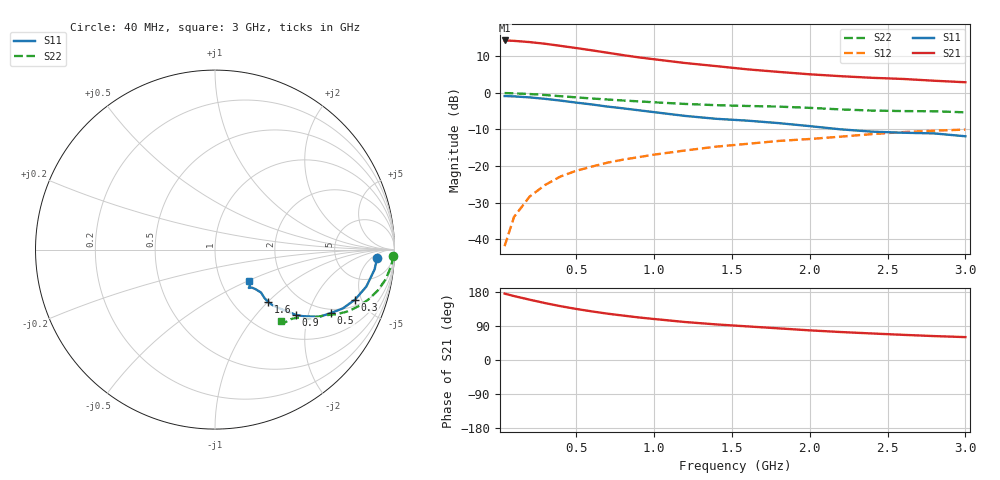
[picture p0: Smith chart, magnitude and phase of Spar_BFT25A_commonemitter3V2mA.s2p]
! Filename:  BFT25AJ.S2P  Version:  2.0
! NXP part #: BFT25A  Date: Aug 1990
! Bias condition: Vce=3V, Ic=2mA
#  MHz  S  MA  R  50
! Freq  S11  S21  S12  S22  !GUM [dB]
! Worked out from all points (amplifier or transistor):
!   21 points, 40 MHz to 3 GHz, reference 50 ohm
!   highest |S21| = 14.3 dB at 40 MHz (marker M1)
!   |S21| within 3 dB of that: start of sweep to 646.2 MHz
!   unconditionally stable (mu >= 1): 1.946 GHz to end of sweep
!   at 300 MHz: K = 0.31, MSG = 19.3 dB, |S12| = -25.2 dB
!   at 1 GHz: K = 0.76, MSG = 13.0 dB, |S12| = -16.9 dB
!   at 3 GHz: K = 1.09, MAG = 4.6 dB, |S12| = -10.0 dB
!   S11 on the Smith chart (normalised r, x): 40 MHz: 16, -8; 300 MHz: 2.50, -4.44; 500 MHz: 1.83, -2.82; 900 MHz: 1.53, -1.68; 1.6 GHz: 1.43, -1.01; 3 GHz: 1.35, -0.50
40  0.905 -2.9  5.215 175.2  0.008 86.7  0.994 -2.0
100  0.896 -7.1  5.152 168.8  0.02 84.5  0.987 -5.1
200  0.868 -13.7  4.955 159.3  0.038 81.9  0.965 -9.9
300  0.829 -19.6  4.7 150.2  0.055 78.2  0.935 -14.1
400  0.784 -24.7  4.396 142.0  0.072 75.9  0.901 -17.8
500  0.736 -28.7  4.105 134.7  0.086 73.0  0.869 -20.8
600  0.695 -32.5  3.824 128.3  0.098 71.6  0.838 -23.2
700  0.65 -35.0  3.544 122.3  0.111 70.2  0.812 -25.2
800  0.615 -37.1  3.287 117.3  0.122 69.0  0.787 -26.7
900  0.579 -38.9  3.066 112.4  0.132 68.3  0.766 -28.1
1000  0.545 -40.0  2.884 108.2  0.143 67.6  0.744 -29.1
1200  0.484 -42.4  2.561 100.2  0.163 65.8  0.706 -31.4
1400  0.442 -44.1  2.323 93.9  0.184 64.8  0.679 -33.7
1600  0.417 -44.5  2.099 88.7  0.201 63.9  0.662 -35.1
1800  0.386 -44.4  1.937 83.5  0.22 63.1  0.649 -36.6
2000  0.351 -43.0  1.796 78.2  0.234 61.4  0.624 -37.6
2200  0.317 -44.2  1.692 73.8  0.252 59.8  0.594 -39.6
2400  0.295 -45.8  1.608 70.0  0.273 58.7  0.573 -42.6
2600  0.285 -48.6  1.551 66.4  0.291 57.4  0.564 -45.6
2800  0.279 -46.0  1.466 63.1  0.304 56.7  0.56 -46.7
3000  0.255 -42.9  1.398 60.4  0.315 56.0  0.542 -47.3
